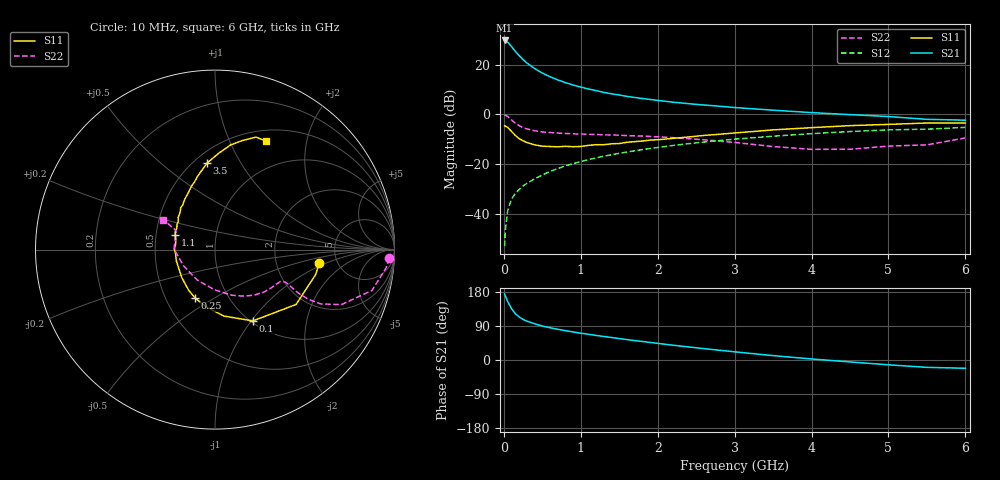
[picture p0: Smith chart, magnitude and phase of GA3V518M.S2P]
! Infineon Technologies  Discrete & RF Semiconductors
! BF775
! Si NPN RF Bipolar Junction Transistor in SOT23
! VCE = 3.5 V  IC = 18 mA
! Common Emitter S-Parameters:  May  1996
# GHz  S  MA  R  50
!  f  S11  S21  S12  S22
! GHz  MAG  ANG  MAG  ANG  MAG  ANG  MAG  ANG
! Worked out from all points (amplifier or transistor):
!   36 points, 10 MHz to 6 GHz, reference 50 ohm
!   highest |S21| = 29.7 dB at 10 MHz (marker M1)
!   |S21| within 3 dB of that: start of sweep to 113.8 MHz
!   unconditionally stable (mu >= 1): 407.7 MHz to 3.127 GHz
!   at 250 MHz: K = 0.84, MSG = 25.4 dB, |S12| = -28.9 dB
!   at 1.4 GHz: K = 1.11, MAG = 10.2 dB, |S12| = -16.3 dB
!   at 6 GHz: K = 0.95, MSG = 1.5 dB, |S12| = -5.3 dB
!   S11 on the Smith chart (normalised r, x): 10 MHz: 3.62, -0.82; 100 MHz: 1.02, -1.02; 250 MHz: 0.70, -0.41; 1.1 GHz: 0.63, +0.11; 3.5 GHz: 0.58, +0.73; 6 GHz: 0.63, +1.38
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0.01  0.5851 -7.3  30.68 174.4  0.0022 90.1  0.9725 -2.9
0.02  0.5782 -13.8  30.27 169.0  0.0047 82.3  0.9581 -6.2
0.05  0.5453 -34.1  28.31 154.3  0.0114 76.4  0.9035 -14.6
0.1  0.4498 -62.0  23.12 135.4  0.0195 68.5  0.7683 -23.5
0.15  0.3734 -82.4  18.45 122.1  0.0256 65.1  0.6619 -27.2
0.2  0.3223 -98.9  15.09 113.5  0.0306 65.6  0.5888 -28.0
0.25  0.2921 -112.1  12.59 107.2  0.0359 65.6  0.5374 -27.7
0.3  0.2702 -122.8  10.79 102.4  0.0406 66.8  0.5062 -27.2
0.4  0.2419 -140.0  8.346 95.6  0.05 68.1  0.4655 -25.8
0.5  0.2271 -153.1  6.762 89.7  0.0598 69.2  0.4402 -25.0
0.6  0.2242 -164.0  5.707 85.2  0.0703 69.3  0.4283 -24.9
0.7  0.2208 -173.2  4.939 81.1  0.0805 69.3  0.4184 -25.2
0.8  0.2262 179.9  4.343 77.4  0.0911 69.0  0.4107 -25.7
0.9  0.2217 172.7  3.886 73.9  0.1015 68.5  0.4036 -26.2
1.1  0.2359 160.2  3.234 68.0  0.1219 67.4  0.3944 -28.8
1.3  0.2437 151.0  2.76 62.1  0.1427 65.6  0.3856 -31.5
1.6  0.2729 138.9  2.288 53.7  0.1735 62.9  0.3713 -36.1
2.2  0.327 121.1  1.752 39.0  0.2348 56.5  0.3379 -48.0
3.5  0.4843 95.2  1.208 11.5  0.3613 40.1  0.2238 -90.8
4.5  0.5898 81.5  0.983 -5.1  0.4489 26.7  0.1972 -152.5
5.5  0.6669 70.0  0.79 -19.4  0.5005 11.7  0.2419 153.8
6  0.6679 64.9  0.76 -21.8  0.5439 7.6  0.3333 149.9
